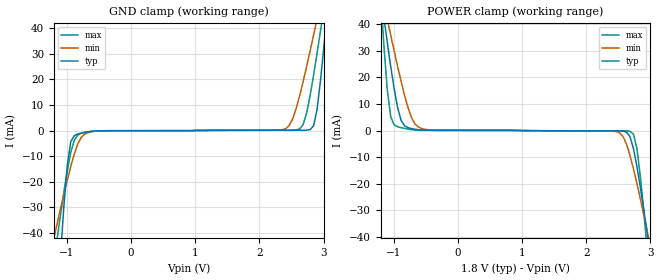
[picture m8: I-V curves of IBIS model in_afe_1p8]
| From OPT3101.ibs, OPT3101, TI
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|   afe_in_1p8 Model
[Model]   in_afe_1p8
Model_type   Input
Vinl = 0.54
Vinh = 1.26
|   typ   min   max
|   (nom PVT)   (fast PVT)   (slow PVT)
C_comp   2.094e-12   1.903e-12   2.287e-12
[Model spec]
|subparameter
| Where nom  PVT is Nominal Process, 1.8V, 27C
|   Fast PVT is Strong Process,  1.9V, -40C
|   Slow PVT is Weak Process,   1.7V, 125C
[Voltage Range]   1.8   1.7   1.9
|Junction Temperature
[Temperature Range]   27   125   -40
[Power Clamp Reference]   1.8   1.7   1.9
[GND Clamp Reference]   0   0   0
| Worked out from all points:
|   GND clamp passes 1 mA (typ) near -0.77 V on its own axis
|   POWER clamp passes 1 mA (typ) near -0.76 V on its own axis
[GND Clamp]
|   Voltage   I(typ)   I(min)   I(max)
-1.8V     -360.3mA   -114mA     -167.4mA
-1.206V   -94.15mA   -42.93mA   -52.66mA
-1.098V   -49.81mA   -30.76mA   -33.26mA
-936mV    -4.353mA   -13.97mA   -8.559mA
-828mV    -1.356mA   -5.319mA   -1.78mA
2.412V    118.3uA    732.4uA    117.3uA
2.682V    128.8uA    19.14mA    2.363mA
2.79V     347.4uA    31.02mA    13.59mA
2.898V    8.133mA    43.53mA    30.01mA
2.952V    19.44mA    49.93mA    38.89mA
3.06V     47.63mA    62.9mA     57.29mA
3.6V      207.3mA    129.7mA    153.7mA
[POWER Clamp]
|   Voltage   I(typ)   I(min)   I(max)
-1.8V     167mA      126mA      315mA
-1.206V   52.7mA     54.5mA     53mA
-1.152V   42.8mA     48.2mA     32.6mA
-1.044V   24.1mA     35.9mA     5.14mA
-936mV    8.56mA     24mA       1.42mA
-720mV    719uA      4.84mA     333uA
-558mV    180uA      738uA      101uA
2.466V    -121uA     -353uA     -123uA
2.682V    -2.36mA    -9.37mA    -287uA
2.79V     -13.6mA    -20mA      -6.81mA
2.952V    -38.9mA    -38.2mA    -45.4mA
3.6V      -154mA     -117mA     -238mA
